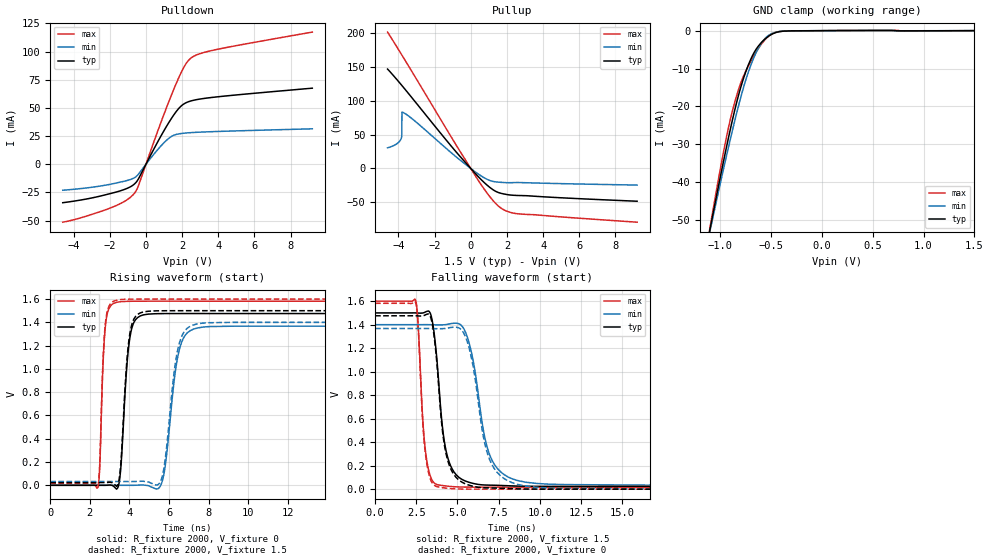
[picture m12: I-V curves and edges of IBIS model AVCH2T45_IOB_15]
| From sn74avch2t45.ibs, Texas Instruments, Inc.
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[Model]   AVCH2T45_IOB_15
Model_type  I/O
Vinl=0.49
Vinh=1.04
Enable   Active-High
Vref =   0
Rref =   2000
Cref =   15p
Vmeas =   0.75
| variable   typ   min   max
C_comp   5.29pF   4.65pF   5.89pF
| C_pullup   5.23pF   3.72pF   7.65pF
| C_pulldown   4.92pF   4.34pF   5.58pF
| C_tri-state   5.29pF   4.65pF   5.89pF
[Temperature Range]   40   100   -40
| Ambient temperature   25   85   -40
[Voltage range]   1.5   1.4   1.6
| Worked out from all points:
|   slope of the pulldown table from 0 to 0.225 V, typ, clamps not added: 32.1 ohm
|   slope of the pullup table from 0 to 0.225 V, typ, clamps not added: 33.9 ohm
|   GND clamp passes 1 mA (typ) near -0.50 V on its own axis
|   rising waveform, R_fixture 2000, V_fixture 0: 20-80 % time 334ps typ, 543ps min, 203ps max; typ from 0 V to 1.48 V
|   falling waveform, R_fixture 2000, V_fixture 1.5: 20-80 % time 638ps typ, 1.02ns min, 392ps max; typ from 1.5 V to 0.023 V
|   rising waveform, R_fixture 2000, V_fixture 1.5: 20-80 % time 330ps typ, 531ps min, 201ps max; typ from 0.023 V to 1.5 V
|   falling waveform, R_fixture 2000, V_fixture 0: 20-80 % time 639ps typ, 1.01ns min, 387ps max; typ from 1.48 V to 0 V
[GND Clamp]
| AVCH2T45_IOB_15
|   Voltage   I(typ)   I(min)   I(max)
-4.6V     -599.6mA   -548.2mA   -664.6mA
-1.1V     -52.36mA   -52.8mA    -51.85mA
-1.075V   -48.9mA    -49.67mA   -47.95mA
-930mV    -29.68mA   -32.07mA   -27.01mA
-880mV    -23.6mA    -26.34mA   -21.2mA
-830mV    -18.08mA   -20.9mA    -16.41mA
-765mV    -12.13mA   -14.48mA   -11.64mA
-685mV    -6.738mA   -8.147mA   -7.41mA
-605mV    -3.434mA   -3.729mA   -3.946mA
-535mV    -1.679mA   -1.475mA   -1.741mA
-370mV    -121.9uA   -99.54uA   -128.4uA
1.5V      812.2pA    1.554uA    -44.11nA
[Pulldown]
| AVCH2T45_IOB_15
|   Voltage   I(typ)   I(min)   I(max)
-4.6V     -34.07mA   -23.01mA   -51.35mA
-1.88V    -25.6mA    -17.43mA   -38.2mA
-1.09V    -21.68mA   -14.59mA   -31.97mA
-625mV    -17.31mA   -11.83mA   -25.44mA
-415mV    -12.94mA   -8.777mA   -18.95mA
595mV     18.22mA    11.97mA    26.91mA
1.265V    37.01mA    23.01mA    55.56mA
1.695V    47.18mA    26.54mA    72.43mA
2.025V    52.71mA    27.44mA    83.88mA
2.495V    56.22mA    28.09mA    94.25mA
3.835V    59.62mA    29.04mA    101.6mA
9.2V      67.51mA    31.46mA    117.2mA
[Pullup]
| AVCH2T45_IOB_15
|   Voltage   I(typ)   I(min)   I(max)
-4.6V     146.8mA    30.47mA    201.5mA
-4.1V     131.8mA    36.24mA    180.2mA
-3.85V    123.9mA    43.97mA    169.4mA
-3.81V    122.6mA    49.37mA    167.6mA
-3.805V   122.5mA    83.3mA     167.4mA
-3.785V   121.8mA    83.17mA    166.5mA
-3.155V   101.3mA    71.56mA    138.9mA
175mV     -5.197mA   -3.574mA   -7.497mA
980mV     -26.35mA   -16.94mA   -39.04mA
1.625V    -36.35mA   -20.39mA   -57.65mA
2.595V    -39.89mA   -20.78mA   -66.9mA
9.2V      -48.41mA   -24.54mA   -79.36mA
[Ramp]
| AVCH2T45_IOB_15
| variable   typ   min   max
dV/dt_r   0.91/3.44E-10   0.84/5.58E-10   0.96/2.08E-10
dV/dt_f   0.90/6.47E-10   0.83/1.02E-09   0.96/3.97E-10
R_load = 2000
[Rising Waveform]
| AVCH2T45_IOB_15
R_fixture =   2000
C_fixture =   0
L_fixture =   0
V_fixture =   0
V_fixture_min = 0
V_fixture_max = 0
|   Time   V(typ)   V(min)   V(max)
0s        19.41nV    97.7nV     527.2pV
2.425ns   23.6uV     1.698uV    -13.39mV
2.785ns   -46.51uV   -12.06uV   1.368V
3.35ns    -33.32mV   10.91uV    1.572V
4.015ns   1.261V     -140uV     1.581V
4.705ns   1.464V     2.618mV    1.582V
5.64ns    1.475V     25.2mV     1.582V
6.49ns    1.476V     1.144V     1.582V
7.425ns   1.476V     1.351V     1.582V
40ns      1.476V     1.367V     1.582V
[Falling Waveform]
| AVCH2T45_IOB_15
R_fixture =   2000
C_fixture =   0
L_fixture =   0
V_fixture =   1.5
V_fixture_min = 1.4
V_fixture_max = 1.6
|   Time   V(typ)   V(min)   V(max)
0s        1.5V       1.4V       1.6V
2.46ns    1.5V       1.4V       1.607V
3.065ns   1.509V     1.4V       317.1mV
3.785ns   1.05V      1.398V     38.58mV
4.2ns     409.6mV    1.399V     28.86mV
4.78ns    148.2mV    1.412V     20.96mV
5.71ns    58.08mV    1.242V     17.52mV
6.985ns   34.11mV    281.4mV    17.14mV
8.63ns    26.54mV    73.97mV    17.11mV
40ns      23.4mV     32.34mV    17.1mV
[Rising Waveform]
| AVCH2T45_IOB_15
R_fixture =   2000
C_fixture =   0
L_fixture =   0
V_fixture =   1.5
V_fixture_min = 1.4
V_fixture_max = 1.6
|   Time   V(typ)   V(min)   V(max)
0s        23.4mV     32.34mV    17.1mV
2.425ns   23.42mV    32.34mV    4.425mV
2.78ns    23.33mV    32.32mV    1.385V
3.34ns    -7.585mV   32.35mV    1.59V
4.01ns    1.292V     32.2mV     1.599V
4.69ns    1.489V     34.86mV    1.6V
5.62ns    1.499V     55.41mV    1.6V
6.46ns    1.5V       1.18V      1.6V
7.39ns    1.5V       1.385V     1.6V
40ns      1.5V       1.4V       1.6V
[Falling Waveform]
| AVCH2T45_IOB_15
R_fixture =   2000
C_fixture =   0
L_fixture =   0
V_fixture =   0
V_fixture_min = 0
V_fixture_max = 0
|   Time   V(typ)   V(min)   V(max)
0s        1.476V     1.367V     1.582V
2.46ns    1.476V     1.367V     1.588V
3.06ns    1.484V     1.367V     297.3mV
3.785ns   1.016V     1.366V     20.92mV
4.195ns   385.6mV    1.367V     10.84mV
4.78ns    124.9mV    1.378V     3.296mV
5.695ns   34.51mV    1.208V     369.6uV
6.94ns    10.69mV    256mV      39.52uV
8.62ns    2.823mV    41.57mV    7.909uV
40ns      368.4nV    636.3nV    219.5nV
